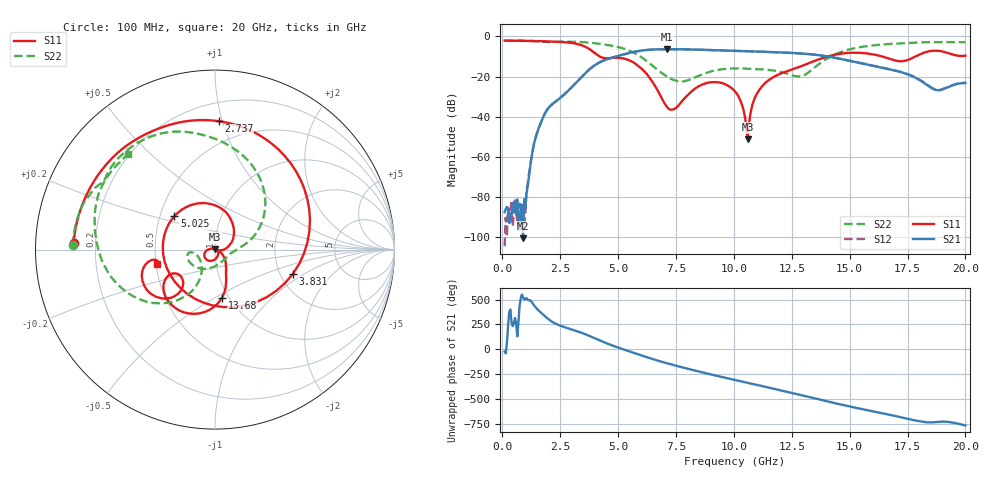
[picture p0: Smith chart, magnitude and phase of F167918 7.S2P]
!  2-Port S-parameters saved by WinCal
! VAR MeasName=S-Parameters (CALIBRATED_DATA) read from VNA (N5242A)
! VAR MeasDate=2016-11-22 10:25:10
! VAR NAME=F167918 7
! VAR FILENAME=F167918 7.S2P
! VAR DATE=2016-11-22 10:25:10
! VAR PHYS_PORTS=1,2
# Hz S DB R 50
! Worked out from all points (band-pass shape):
!   401 points, 100 MHz to 20 GHz, reference 50 ohm
!   highest |S21| = -6.35 dB at 7.115 GHz (marker M1); lowest = -100.6 dB at 896 MHz (marker M2)
!   |S21| within 3 dB of the highest: 5.102 GHz to 13.67 GHz (8.567 GHz wide, 91.3 % of centre)
!   lowest |S11| = -51.3 dB at 10.6 GHz (marker M3), VSWR 1.01, Z = 50.1 + j0.237 ohm
!   |S11| at or under -10 dB: 4.213 GHz to 14.03 GHz (9.822 GHz wide, 108 % of centre); 16.4 GHz to 17.84 GHz (1.433 GHz wide, 8.37 % of centre)
!   |S22| runs from -22.5 to -2.0 dB; largest |S21 - S12| = 0.004
!   S11 on the Smith chart (normalised r, x): 100 MHz: 0.12, +0.02; 2.737 GHz: 0.33, +0.97; 3.831 GHz: 2.34, -0.80; 5.025 GHz: 0.59, +0.24; 13.68 GHz: 0.93, -0.54; 20 GHz: 0.51, -0.09
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1e8  -2.07 177.3  -87.54 -25.8  -104.46 116.0  -2.00 178.3
8.96e8  -2.19 156.0  -100.58 165.2  -86.77 -38.2  -2.11 165.0
1.692e9  -2.36 132.1  -42.16 3.1  -42.07 2.3  -2.54 151.7
2.73675e9  -2.90 88.3  -28.25 -142.4  -28.24 -142.7  -2.60 135.9
3.43325e9  -4.40 34.4  -20.09 163.9  -20.12 163.8  -2.79 120.0
3.83125e9  -6.86 -17.4  -15.76 126.1  -15.75 126.1  -3.14 109.3
4.478e9  -10.85 -140.9  -11.58 61.1  -11.53 60.8  -4.14 90.9
5.02525e9  -10.66 140.6  -9.61 14.1  -9.61 13.6  -5.34 72.2
5.9705e9  -15.61 52.1  -7.10 -60.6  -7.13 -60.8  -10.06 32.0
6.7665e9  -28.15 -4.5  -6.40 -119.4  -6.42 -119.4  -17.16 4.2
7.11475e9  -35.07 -12.9  -6.35 -142.7  -6.37 -142.7  -20.00 -7.3
8.856e9  -23.09 -116.3  -6.72 113.2  -6.71 113.2  -17.96 -122.7
1.005e10  -27.42 -177.5  -7.17 48.8  -7.18 48.9  -15.97 -160.0
1.059725e10  -51.28 60.0  -7.38 20.3  -7.39 20.2  -16.10 -167.7
1.089575e10  -30.77 -22.7  -7.50 4.7  -7.49 4.7  -16.22 -169.9
1.129375e10  -23.84 -39.6  -7.64 -16.3  -7.64 -16.1  -16.49 -172.5
1.338325e10  -12.65 -76.0  -8.95 -129.6  -8.90 -129.2  -16.49 -120.2
1.368175e10  -11.35 -81.8  -9.37 -146.5  -9.32 -146.1  -13.74 -117.1
1.51245e10  -8.10 -121.2  -12.46 136.3  -12.37 136.4  -6.09 -145.4
1.67165e10  -11.10 -151.0  -16.34 58.7  -16.32 58.8  -3.79 -179.0
1.875625e10  -7.12 -154.9  -26.72 -15.0  -26.55 -15.3  -2.81 148.6
2e10  -9.59 -166.4  -23.16 -49.2  -23.01 -49.8  -2.86 132.5
